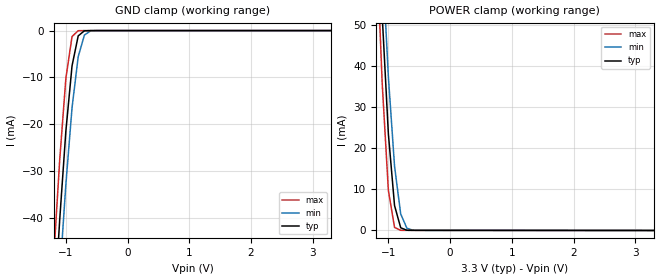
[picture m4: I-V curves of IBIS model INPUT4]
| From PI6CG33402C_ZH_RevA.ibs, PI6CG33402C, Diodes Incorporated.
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[Model] INPUT4
Model_type Input
Vinl = 825mV
Vinh = 2.75V
| variable   typ   min   max
C_comp   0.443pF   0.441pF   0.445pF
[Voltage Range]   3.3V   3.135V   3.465V
[GND Clamp Reference]   0.000V   0.000V   0.000V
[POWER Clamp Reference]   3.3V   3.135V   3.465V
[temperature range]   25   85   -40
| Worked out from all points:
|   GND clamp passes 1 mA (typ) near -0.79 V on its own axis
|   POWER clamp passes 1 mA (typ) near -0.81 V on its own axis
[GND Clamp]
| Voltage   I(typ)   I(min)   I(max)
-3.3V     -611mA     -617mA     -607mA
-1.2V     -62.2mA    -74.3mA    -49.3mA
-1.1V     -40.5mA    -52.6mA    -27.7mA
-1V       -21.5mA    -32.9mA    -10.2mA
-900mV    -7.54mA    -16.5mA    -1.27mA
-800mV    -1.13mA    -5.57mA    -24.2uA
-700mV    -53.2uA    -958uA     -202nA
-600mV    -1.35uA    -74.3uA    -1.53nA
3.3V      9.9pA      35.5pA     9.41pA
[POWER Clamp]   |Note: Vtable = Vcc - Voutput
| Voltage   I(typ)   I(min)   I(max)
-3.3V     1.03A      987mA      1.09A
-1.2V     87.7mA     101mA      72.8mA
-1.1V     52.3mA     66.8mA     35.8mA
-1V       23.5mA     37.4mA     9.72mA
-900mV    6.04mA     15.6mA     710uA
-800mV    623uA      3.98mA     15.5uA
-700mV    27.9uA     521uA      5.41uA
-600mV    5.47uA     38.2uA     4.57uA
3.3V      -27.3uA    -28.7uA    -25.2uA
